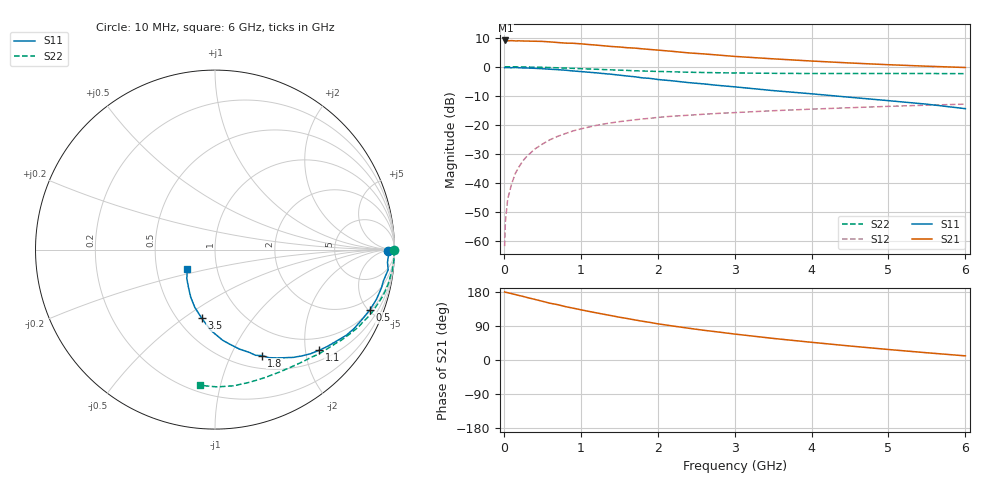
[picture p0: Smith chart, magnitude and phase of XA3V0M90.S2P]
! SIEMENS Discrete & RF Semiconductors
! BFY180
! Si NPN RF Bipolar Junction Transistor in MICRO-X
! VCE = 3 V  IC = 0.9 mA
! Common Emitter S-Parameters:  May  1997
# GHz  S  MA  R  50
!  f  S11  S21  S12  S22
! GHz  MAG  ANG  MAG  ANG  MAG  ANG  MAG  ANG
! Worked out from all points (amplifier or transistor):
!   36 points, 10 MHz to 6 GHz, reference 50 ohm
!   highest |S21| = 9.1 dB at 20 MHz (marker M1)
!   |S21| within 3 dB of that: start of sweep to 1.851 GHz
!   unconditionally stable (mu >= 1): 3.991 GHz to end of sweep
!   at 250 MHz: K = 0.06, MSG = 20.6 dB, |S12| = -32.4 dB
!   at 1.4 GHz: K = 0.49, MSG = 13.2 dB, |S12| = -19.3 dB
!   at 6 GHz: K = 1.06, MAG = 4.8 dB, |S12| = -12.9 dB
!   S11 on the Smith chart (normalised r, x): 10 MHz: 55, -11; 500 MHz: 1.08, -5.10; 1.1 GHz: 0.71, -2.28; 1.8 GHz: 0.65, -1.32; 3.5 GHz: 0.65, -0.59; 6 GHz: 0.72, -0.16
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0.01  0.9653 -0.4  2.82 179.6  0.0008 83.0  0.9984 -0.2
0.02  0.9662 -0.8  2.848 178.8  0.0021 84.5  0.9999 -0.6
0.05  0.9666 -2.1  2.804 177.6  0.0052 84.7  0.9973 -1.3
0.1  0.9637 -4.2  2.83 175.2  0.0094 89.7  0.9986 -2.6
0.15  0.9713 -6.7  2.797 172.7  0.0145 84.7  0.9981 -3.9
0.25  0.9539 -10.7  2.787 167.8  0.024 83.5  0.9947 -6.6
0.3  0.9518 -12.9  2.78 165.0  0.0285 80.8  0.9902 -7.8
0.5  0.9259 -21.3  2.744 155.0  0.0462 74.9  0.9793 -12.9
0.6  0.9075 -25.3  2.688 149.8  0.055 72.2  0.9704 -15.3
0.9  0.8471 -37.0  2.546 136.8  0.0781 63.5  0.9398 -22.2
1.1  0.8068 -44.1  2.426 128.5  0.0908 58.9  0.9166 -26.3
1.5  0.7174 -57.1  2.197 113.0  0.1129 50.5  0.8752 -34.0
1.8  0.6448 -66.3  2.044 102.3  0.1256 45.9  0.8464 -39.0
2  0.6042 -71.5  1.942 95.5  0.1338 42.5  0.8317 -42.2
2.2  0.5707 -76.2  1.843 89.6  0.1405 39.7  0.82 -45.2
2.6  0.5059 -85.3  1.668 78.4  0.1517 35.3  0.7968 -50.7
3  0.4505 -93.0  1.511 68.5  0.1618 31.2  0.7819 -56.0
3.5  0.3881 -101.1  1.372 57.0  0.1744 27.0  0.7711 -62.3
4  0.3415 -109.2  1.257 46.7  0.1857 22.8  0.7654 -68.7
4.5  0.2977 -117.0  1.163 36.9  0.1965 19.0  0.764 -75.3
5.5  0.226 -134.0  1.023 19.1  0.2175 11.0  0.7651 -89.1
6  0.1892 -145.0  0.972 10.9  0.2265 6.9  0.7608 -96.1
